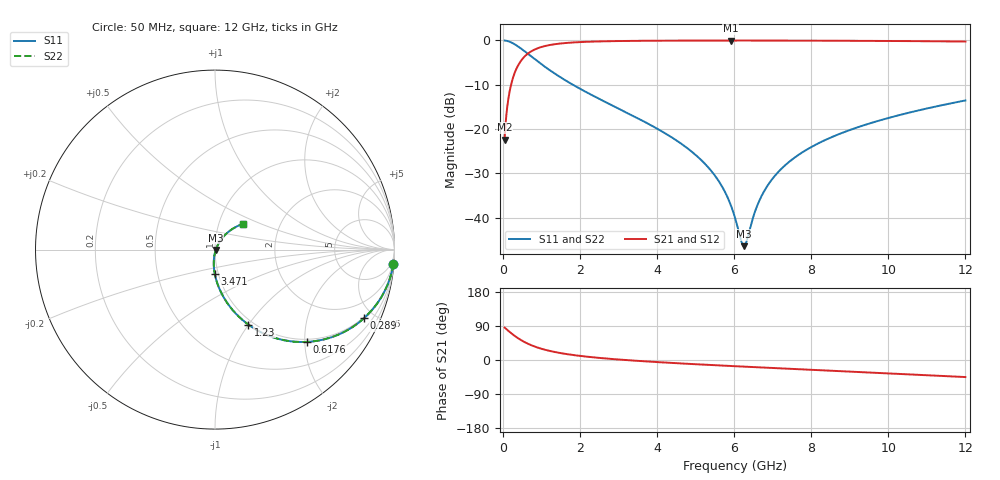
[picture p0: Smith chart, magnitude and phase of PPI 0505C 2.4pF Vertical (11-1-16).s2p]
# GHz S MA R 50
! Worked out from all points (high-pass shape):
!   1601 points, 50 MHz to 12 GHz, reference 50 ohm
!   highest |S21| = -0.04 dB at 5.913 GHz (marker M1); lowest = -22.4 dB at 50 MHz (marker M2)
!   |S21| within 3 dB of the highest: 646.4 MHz to end of sweep
!   lowest |S11| = -46.5 dB at 6.257 GHz (marker M3), VSWR 1.01, Z = 50.5 - j0.148 ohm
!   |S11| at or under -10 dB: 1.817 GHz to end of sweep
!   |S22| runs from -46.5 to 0.0 dB; largest |S21 - S12| = 0
!   S11 on the Smith chart (normalised r, x): 50 MHz: 1, -25; 289 MHz: 0.94, -4.39; 617.6 MHz: 0.94, -2.04; 1.23 GHz: 0.94, -1.00; 3.471 GHz: 0.96, -0.26; 12 GHz: 1.30, +0.39
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0.05  0.9971 -4.5  0.07596 85.5  0.07596 85.5  0.9971 -4.5
0.1695  0.9681 -15.0  0.2502 75.0  0.2502 75.0  0.9681 -15.0
0.289  0.9147 -24.6  0.4035 65.3  0.4035 65.3  0.9147 -24.6
0.617625  0.7247 -45.2  0.6878 44.7  0.6878 44.7  0.7247 -45.2
0.9014375  0.5807 -56.9  0.8124 33.0  0.8124 33.0  0.5807 -56.9
1.230063  0.4573 -66.0  0.8872 23.7  0.8872 23.7  0.4573 -66.0
2.044156  0.2783 -79.1  0.9577 10.4  0.9577 10.4  0.2783 -79.1
3.470687  0.1341 -90.6  0.9873 -2.1  0.9873 -2.1  0.1341 -90.6
4.038312  0.09883 -93.5  0.9911 -5.7  0.9911 -5.7  0.09883 -93.5
5.24825  0.04028 -96.3  0.9946 -12.4  0.9946 -12.4  0.04028 -96.3
5.629156  0.02472 -94.0  0.9949 -14.4  0.9949 -14.4  0.02472 -94.0
5.912969  0.0139 -86.5  0.9949 -15.8  0.9949 -15.8  0.0139 -86.5
6.025  0.009953 -78.6  0.9949 -16.4  0.9949 -16.4  0.009953 -78.6
6.181844  0.005505 -48.3  0.9949 -17.1  0.9949 -17.1  0.005505 -48.3
6.256531  0.004746 -18.0  0.9949 -17.5  0.9949 -17.5  0.004746 -18.0
6.32375  0.005376 9.5  0.9948 -17.8  0.9948 -17.8  0.005376 9.5
6.615031  0.01407 50.3  0.9946 -19.3  0.9946 -19.3  0.01407 50.3
6.906313  0.02421 57.3  0.9942 -20.7  0.9942 -20.7  0.02421 57.3
7.376844  0.04068 59.7  0.9935 -22.9  0.9935 -22.9  0.04068 59.7
8.019156  0.06297 59.0  0.992 -25.9  0.992 -25.9  0.06297 59.0
10.01331  0.1333 51.8  0.9839 -35.3  0.9839 -35.3  0.1333 51.8
12  0.2096 42.9  0.9694 -45.0  0.9694 -45.0  0.2096 42.9
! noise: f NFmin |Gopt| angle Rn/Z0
0.05  0.0007322  0.9404  1.93  0.002742
1.372  0.0057  0.7612  4.866  0.004831
2.701  0.00925  0.7171  8.271  0.006431
4.031  0.01242  0.6909  11.74  0.00774
5.36  0.01542  0.6733  15.2  0.008937
6.682  0.01833  0.6614  18.61  0.0101
8.012  0.02128  0.6536  21.98  0.01129
9.341  0.02429  0.6492  25.3  0.01254
10.67  0.02741  0.6477  28.55  0.0139
12  0.03071  0.6488  31.76  0.01541
